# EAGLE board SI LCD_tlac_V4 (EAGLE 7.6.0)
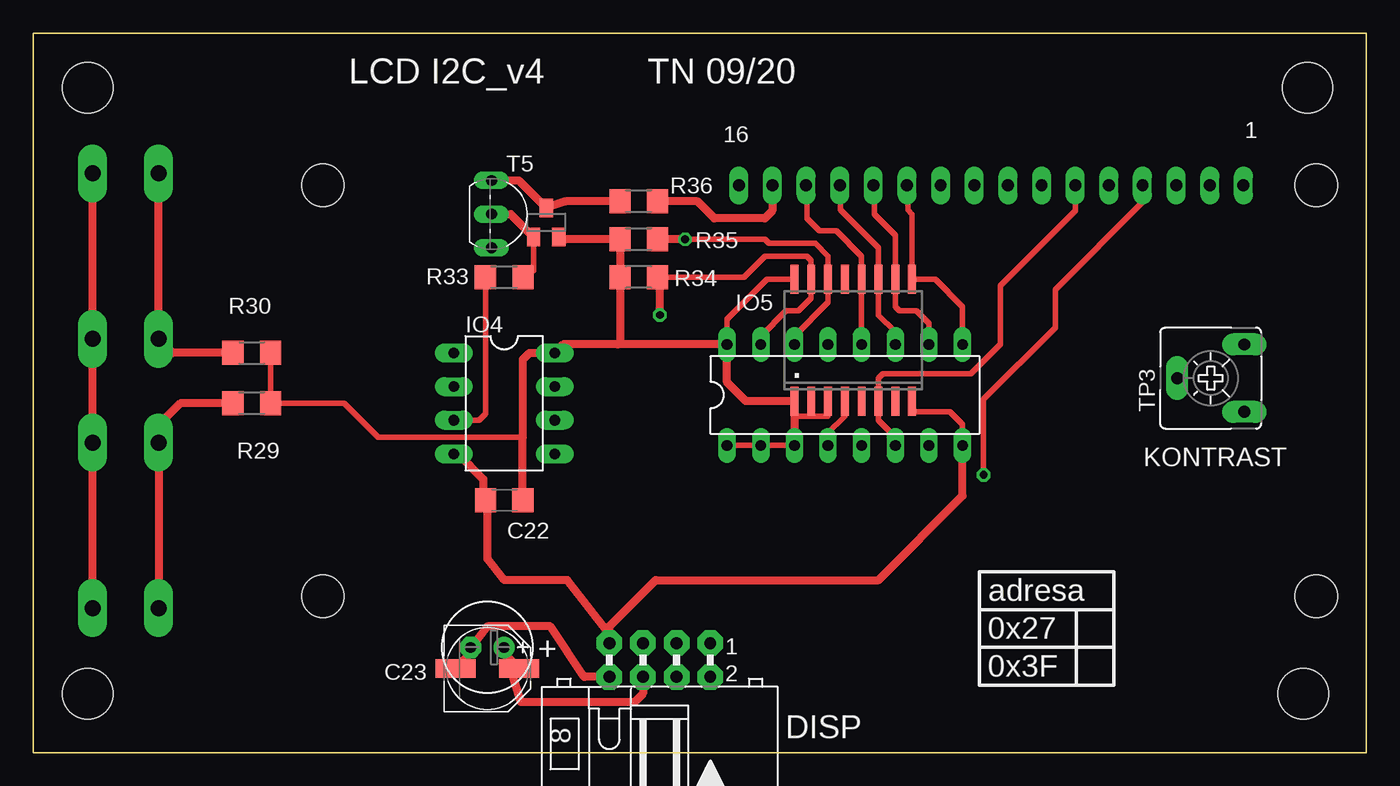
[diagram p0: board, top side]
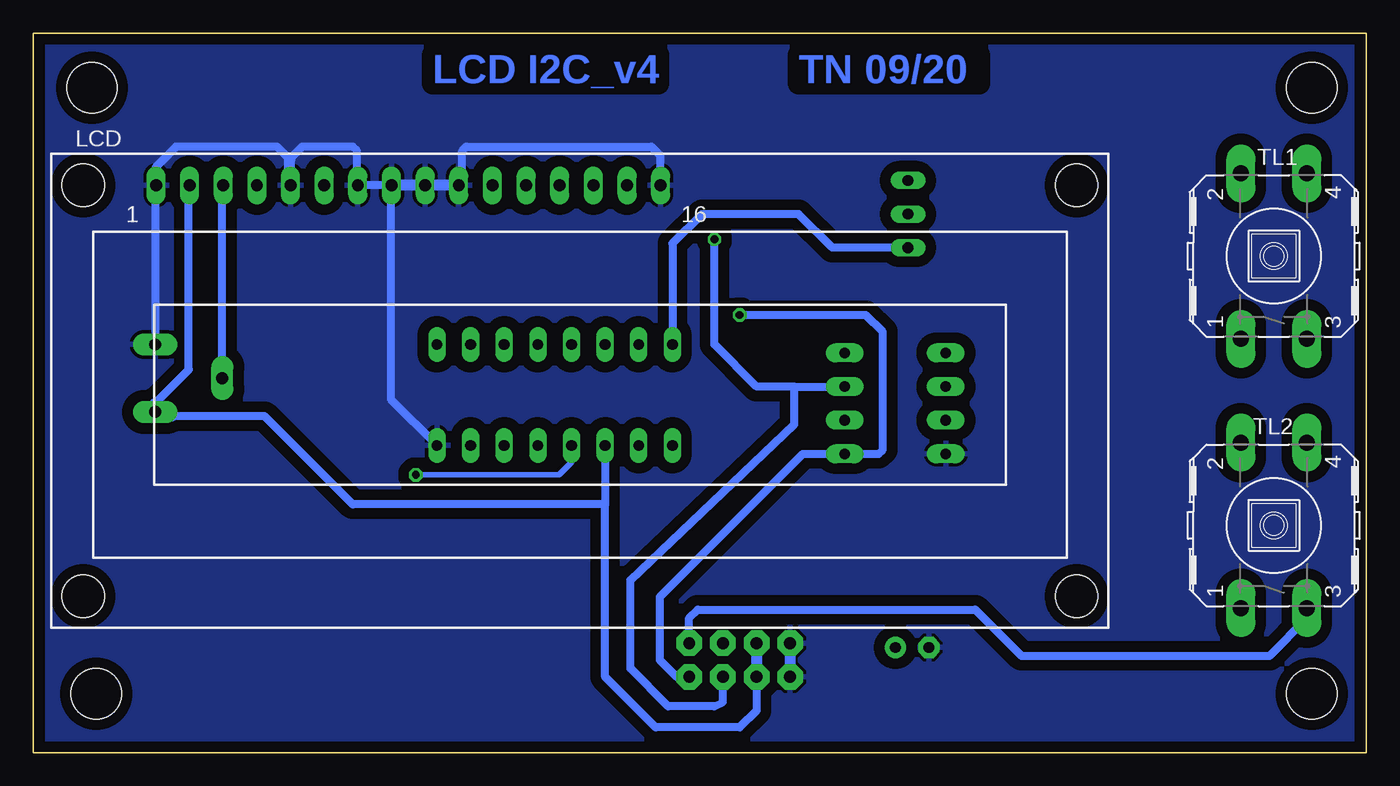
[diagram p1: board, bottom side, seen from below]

Size 100.65 x 54.29 mm. Coordinates in mm from the lower left corner, seen from the top.
Outline: 0,54.29 100.65,54.29 100.65,0 0,0 0,54.29
Copper layers (1*16): Top 0.035mm / dielectric 1.5mm / Bottom 0.035mm
Design rules "default *": minimum track width 10mil, minimum drill 24mil, track to track 8mil, track to pad 8mil, pad to pad 8mil, via to via 8mil, smd to smd 8mil, copper to edge 20mil, drill to drill 8mil, minimum pad ring 10mil, minimum via ring 8mil, stop-mask expansion 4mil, vias tented up to drill 0mil, thermal gap 10mil
Holes 3.8 mm at 4.13,4.45 4.13,50.16 96.2,50.16 95.89,4.45

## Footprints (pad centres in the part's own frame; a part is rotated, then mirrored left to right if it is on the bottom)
C1206 = smd 1.6 x 1.8: 1 -1.4,0; 2 1.4,0
E2,5-7 = drill 0.813 pad 1.6: + -1.27,0 | drill 0.813 pad 1.6 octagon: - 1.27,0
PANASONIC_D = smd 3 x 1.4: + 2.4,0; - -2.4,0
ML8L = drill 0.9 pad 1.93 octagon: 1 -5.08,-2.54; 2 -5.08,0; 3 -2.54,-2.54; 4 -2.54,0; 5 0,-2.54; 6 0,0; 7 2.54,-2.54; 8 2.54,0
DIL16 = drill 0.813 long: 1 -8.89,-3.81; 2 -6.35,-3.81; 3 -3.81,-3.81; 4 -1.27,-3.81; 5 1.27,-3.81; 6 3.81,-3.81; 7 6.35,-3.81; 8 8.89,-3.81; 9 8.89,3.81; 10 6.35,3.81; 11 3.81,3.81; 12 1.27,3.81; 13 -1.27,3.81; 14 -3.81,3.81; 15 -6.35,3.81; 16 -8.89,3.81
TO92-CBE = drill 0.813 long: B 0,0; C -2.54,0; E 2.54,0
DIL08 = drill 0.8 pad 1.422 long: 1 -3.81,-3.81; 2 -1.27,-3.81; 3 1.27,-3.81; 4 3.81,-3.81; 5 3.81,3.81; 6 1.27,3.81; 7 -1.27,3.81; 8 -3.81,3.81
SO16W = smd 0.6 x 2.2: 1 -4.445,-4.6; 2 -3.175,-4.6; 3 -1.905,-4.6; 4 -0.635,-4.6; 5 0.635,-4.6; 6 1.905,-4.6; 7 3.175,-4.6; 8 4.445,-4.6; 9 4.445,4.6; 10 3.175,4.6; 11 1.905,4.6; 12 0.635,4.6; 13 -0.635,4.6; 14 -1.905,4.6; 15 -3.175,4.6; 16 -4.445,4.6
TUXGR_16X2_R2 = drill 0.9 pad 1.422 long: 1 -32,15.5; 2 -29.46,15.5; 3 -26.92,15.5; 4 -24.38,15.5; 5 -21.84,15.5; 6 -19.3,15.5; 7 -16.76,15.5; 8 -14.22,15.5; 9 -11.68,15.5; 10 -9.14,15.5; 11 -6.6,15.5; 12 -4.06,15.5; 13 -1.52,15.5; 14 1.02,15.5; 15 3.56,15.5; 16 6.1,15.5 | hole 3.2: -37.5,-15.5; 37.5,-15.5; -37.5,15.5; 37.5,15.5
R1206 = smd 1.6 x 1.803: 1 -1.422,0; 2 1.422,0
SOT23 = smd 1 x 1.4: 1 -0.95,-1.1; 2 0.95,-1.1; 3 0,1.1
RACON12 = drill 1.2 pad 2.184 long: 1 -6.248,2.489; 2 6.248,2.489; 3 -6.248,-2.489; 4 6.248,-2.489
CA6V = drill 0.9 pad 1.676 long: A -2.54,-2.54; E 2.54,-2.54; S 0,2.54

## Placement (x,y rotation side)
C22  100n  [C1206]  35.56,19.05 180 top
C23  47u  [E2,5-7]  34.29,7.94 180 top
C23.  [PANASONIC_D]  34.29,6.35 0 top
DISP  [ML8L]  46.04,5.71 180 top
E$1  [DIL16]  61.28,26.99 0 top
E$2  BC327  [TO92-CBE]  34.61,40.64 270 top
IO4  Attiny x5  [DIL08]  35.56,26.35 270 top
IO5  PCF8574  [SO16W]  61.91,31.11 0 top
LCD  [TUXGR_16X2_R2]  59.37,27.3 0 bottom
R29  10k  [R1206]  16.51,26.35 0 top
R30  5k6  [R1206]  16.51,30.16 180 top
R33  1k  [R1206]  35.56,35.88 180 top
R34  4k7  [R1206]  45.72,35.88 0 top
R35  4k7  [R1206]  45.72,38.73 0 top
R36  100  [R1206]  45.72,41.59 0 top
T5  BC807  [SOT23]  38.73,40.01 0 top
TL1  [RACON12]  6.99,37.47 90 bottom
TL2  [RACON12]  6.99,17.14 90 bottom
TP3  10k  [CA6V]  88.9,28.26 90 top

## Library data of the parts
C22 C23 C23. R29 R30 R33-R36 = rcl
DISP IO4 LCD TL1 TL2 TP3 = 11moje
E$1 = 40xx
E$2 = transistor-neu-to92
IO5 = linear
T5 = transistor

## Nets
GND: C22.2 C23.- C23..- DISP.7 DISP.8 E$1.8 IO4.4 IO5.8 LCD.1 LCD.5 LCD.7 LCD.8 LCD.9 LCD.10 LCD.16 TP3.E
S$1: LCD.3 TP3.S
S$2: E$2.C R36.1 T5.3
S$3: E$2.B R33.1 T5.1
S$6: E$1.4 IO5.4 LCD.4
S$7: DISP.4 E$1.14 IO4.7 IO5.14 R35.2
S$10: E$1.6 IO5.6 LCD.6
S$11: E$1.9 IO5.9 LCD.11
S$12: E$1.10 IO5.10 LCD.12
S$13: E$1.11 IO5.11 LCD.13
S$14: E$1.12 IO5.12 LCD.14
S$15: LCD.15 R36.2
S$16: IO4.3 R33.2
S$20: DISP.2 E$1.15 IO4.5 IO5.15 R34.2
S$21: R30.2 TL1.1 TL1.2
S$22: DISP.1 TL1.3 TL1.4 TL2.3 TL2.4
S$25: R29.1 TL2.1 TL2.2
S$29: IO4.6
VCC: C22.1 C23.+ C23..+ DISP.5 DISP.6 E$1.1 E$1.2 E$1.3 E$1.16 E$2.E IO4.8 IO5.1 IO5.2 IO5.3 IO5.16 LCD.2 R29.2 R30.1 R34.1 R35.1 T5.2 TP3.A

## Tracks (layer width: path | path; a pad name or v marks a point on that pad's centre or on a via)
GND
  Top 0.406: E$1.8 70.17,24.77 69.22,25.72 66.36,25.72 IO5.8
  Top 0.61: IO4.4 32.07,22.54 33.97,20.64 33.97,19.24 C22.2 34.29,18.92 34.29,14.61 35.56,13.02 40.32,13.02 43.5,8.89 DISP.7 43.5,9.53 46.99,13.02 63.82,13.02 70.17,19.37 E$1.8 | DISP.8 41.59,5.71 39.05,9.53 34.29,9.53 33.34,8.26 C23.- 33.02,7.48 C23..-
  Bottom 0.61: 91.44,42.86 TP3.E | LCD.1 91.37,44.2 89.85,45.72 82.23,45.72 81.28,44.77 | LCD.5 81.21,44.84 80.33,45.72 76.52,45.72 76.2,45.4 76.2,42.86 | 73.72,42.8 LCD.7 | 71.12,42.55 71.05,42.61 LCD.9 | 68.26,42.86 68.26,45.4 67.94,45.72 53.98,45.72 53.34,45.09 53.34,42.87 | LCD.10 73.66,42.8 73.66,26.67 E$1.8
  Bottom 0.813: 91.44,42.86 91.38,42.8 LCD.1 | 81.28,44.77 81.28,42.86 81.22,42.8 LCD.5 | 76.2,42.86 76.14,42.8 LCD.7 | 73.72,42.8 73.66,42.86 73.6,42.8 LCD.8 71.18,42.8 71.12,42.86 71.06,42.8 LCD.9 LCD.10 68.32,42.8 | DISP.7 DISP.8 | 53.34,42.87 LCD.16
  pour Bottom (isolate 0.813): 0,0 0,54.29 100.65,54.29 100.65,0
S$1
  Bottom 0.61: TP3.S 86.36,42.86
  Bottom 0.813: 86.36,42.86 86.3,42.8 LCD.3
S$2
  Top 0.61: R36.1 40.17,41.59 T5.3 36.66,43.18 E$2.C
S$3
  Top 0.406: T5.1 37.78,36.36 R33.1
  Top 0.61: E$2.B 36.05,40.64 T5.1
S$6  (via drill 0.6)
  Top 0.406: LCD.4 83.75,41.52 77.15,34.92 77.15,32.07 71.75,26.67 v71.75,20.95 | IO5.4 61.28,25.4 60.01,24.13 E$1.4
  Bottom 0.406: v71.75,20.95 60.96,20.95 60.01,21.91 E$1.4
S$7  (via drill 0.6)
  Top 0.406: v49.21,38.73 55.24,38.73 55.56,38.42 59.05,38.42 60.01,37.47 IO5.14 60.01,33.97 57.47,31.43 E$1.14
  Top 0.61: v49.21,38.73 R35.2
  Bottom 0.61: 43.18,27.62 IO4.7 | DISP.4 48.58,3.81 49.21,3.49 52.7,3.49 55.56,6.35 55.56,13.02 43.18,24.77 43.18,27.62 | 43.18,27.62 46.04,27.62 49.21,30.8 v49.21,38.73
S$10
  Top 0.406: LCD.6 78.67,40.89 73.03,35.24 73.03,30.8 70.8,28.57 64.14,28.57 63.82,28.26 IO5.6 63.82,25.08 65.09,23.81 E$1.6
S$11
  Top 0.406: LCD.11 66.04,42.74 66.04,40.96 66.36,40.64 IO5.9 68.11,35.72 70.17,33.66 E$1.9
S$12
  Top 0.406: LCD.12 63.5,42.74 63.5,40.64 65.09,39.05 IO5.10 65.09,33.66 65.41,33.34 66.67,33.34 67.63,32.38 E$1.10
S$13
  Top 0.406: LCD.13 60.96,42.74 60.96,40.96 63.82,38.1 IO5.11 63.82,33.02 65.09,31.75 E$1.11
S$14
  Top 0.406: LCD.14 58.42,42.74 58.42,40.32 59.37,39.37 60.64,39.37 62.55,37.47 IO5.12 E$1.12
S$15
  Top 0.61: LCD.15 55.81,40.89 55.24,40.32 51.44,40.32 50.16,41.59 R36.2
S$16
  Top 0.406: R33.2 34.14,25.57 33.66,25.08 IO4.3
S$20  (via drill 0.6)
  Top 0.406: R34.2 53.66,35.88 55.24,37.47 58.42,37.47 58.74,37.15 IO5.15 58.74,34.29 57.78,33.34 56.83,33.34 54.93,31.43 E$1.15
  Top 0.61: v47.31,33.02 47.31,35.71 R34.2
  Bottom 0.61: DISP.2 52.07,5.71 53.34,6.99 53.34,11.75 42.55,22.54 IO4.5 38.1,22.54 36.83,22.54 36.51,22.86 36.51,31.75 37.78,33.02 v47.31,33.02
S$21
  Top 0.61: R30.2 10.53,30.16 TL1.1 TL1.2
S$22
  Top 0.61: TL2.3 TL2.4 TL1.3 TL1.4
  Bottom 0.61: DISP.1 51.12,10.16 50.48,10.79 29.53,10.79 26.04,7.3 7.3,7.3 4.45,10.16 4.45,10.85 TL2.3
S$25
  Top 0.61: R29.1 11.11,26.35 9.53,24.77 9.53,23.44 TL2.2 TL2.1
VCC
  Top 0.406: IO5.3 60.01,25.4 58.74,25.4 | IO5.2 58.74,25.4 | 58.74,25.4 57.47,25.4 IO5.1 | E$1.3 E$1.2 E$1.1 | IO5.16 55.4,35.72 52.39,32.7 E$1.16 | R30.1 R29.2 23.5,26.35 26.04,23.81 36.96,23.81
  Top 0.61: E$1.3 IO5.1 53.81,26.52 52.39,27.94 E$1.16 44.13,30.8 | T5.2 40.17,38.73 R35.1 R34.1 44.3,30.96 44.13,30.8 | 44.13,30.8 40.01,30.8 IO4.8 37.47,30.16 36.96,29.66 36.96,23.81 C22.1 | DISP.6 46.04,4.45 45.4,3.81 36.83,3.81 C23.+ 35.88,7.16 C23..+
  Bottom 0.61: 91.44,26.35 88.9,28.89 88.9,42.86 | 90.17,25.4 83.19,25.4 76.52,18.73 57.47,18.73 | DISP.6 46.04,3.17 47.31,1.91 53.66,1.91 57.47,5.71 57.47,18.73 | E$1.3 57.47,18.73 | E$2.E 40.32,38.1 42.86,40.64 50.16,40.64 52.39,38.42 E$1.16
  Bottom 0.813: 91.44,26.35 TP3.A 90.17,25.4 | 88.9,42.86 88.84,42.8 LCD.2 | DISP.5 DISP.6

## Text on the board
Bottom: TN 09/20 | LCD I2C_v4
tNames: LCD I2C_v4 | TN 09/20 | 16 | 1 | . | KONTRAST | adresa | 0x27 | + | 0x3F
